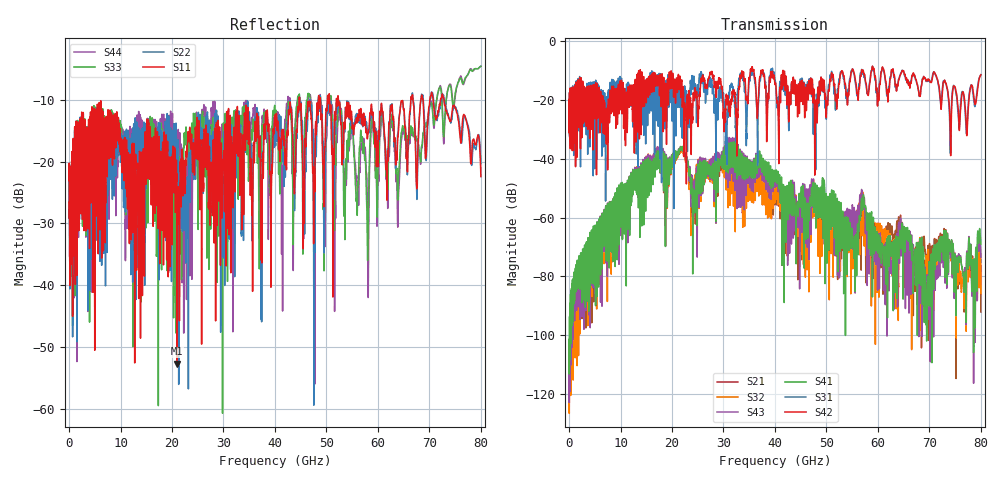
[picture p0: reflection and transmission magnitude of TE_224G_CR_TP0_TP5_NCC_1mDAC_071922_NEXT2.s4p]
!! Reference: tracy_3df_01a_2207
!! CHANNEL DESCRIPTION: TP0_TP5 CR Channel using 1meter DAC, CABLED NCC Host
!! MODEL DESCRIPTION: s4p, NEXT2
!! CONNECTOR DESCRIPTION: OSFP 200G OTB, NCC Socket
!! CABLE DESCRIPTION: 1meter 26AWG Cable
!! MODEL STATUS: Developmental
!! PORT DEFINITIONS:
!! Port  1  ----->  Side A  Side B  <-----  Port  2
!! Port  3  ----->  Side A  Side B  <-----  Port  4
# GHz S MA R 50
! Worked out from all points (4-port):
!   8000 points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, 10 MHz to 80 GHz, reference 50 ohm
!   strongest paths, dB at 10 MHz, 20.01 GHz, 40.01 GHz, 60.01 GHz, 80 GHz:
!     S42: -24.5, -15.0, -14.6, -18.1, -11.4
!     S31: -24.5, -26.1, -13.7, -17.6, -11.4
!     S41: -101.5, -41.7, -47.8, -70.9, -69.0
!     S43: -108.1, -40.8, -48.5, -70.3, -73.5
!     S32: -119.8, -40.8, -53.3, -61.9, -85.9
!     S21: -107.5, -41.6, -55.6, -63.8, -92.1
!   lowest |S11| = -52.7 dB at 21.01 GHz (marker M1), VSWR 1.00, Z = 50 + j0.231 ohm
!   |S11| at or under -10 dB: start of sweep to 44.68 GHz; 52.32 GHz to 66.38 GHz (14.06 GHz wide, 23.7 % of centre); 72.83 GHz to end of sweep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
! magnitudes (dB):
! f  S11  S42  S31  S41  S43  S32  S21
! 10 MHz  -23.1  -24.5  -24.5  -101.5  -108.1  -119.8  -107.5
! 21.01 GHz  -52.7  -16.1  -17.3  -39.0  -38.8  -39.1  -39.4
! 49.32 GHz  -20.4  -15.3  -14.8  -48.9  -46.7  -50.7  -55.6
! 51.89 GHz  -10.5  -18.9  -19.2  -71.1  -71.8  -58.9  -57.8
! 56.84 GHz  -13.9  -9.7  -9.6  -53.4  -50.4  -57.0  -57.9
! 69.36 GHz  -19.0  -13.5  -13.7  -92.3  -81.2  -73.0  -72.6
! 80 GHz  -22.4  -11.4  -11.4  -69.0  -73.5  -85.9  -92.1
